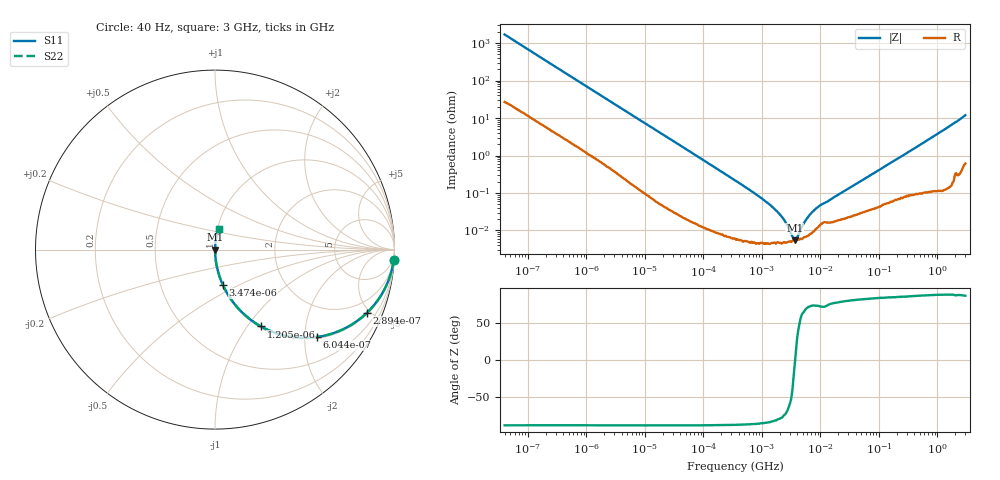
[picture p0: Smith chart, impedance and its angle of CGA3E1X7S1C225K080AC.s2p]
! S-Parameter Data Generated by TDK Corporation
! Copyright(C) 2019 TDK Corporation.
! All Rights Reserved.
! TDK P/N: CGA3E1X7S1C225K080AC (Multilayer Ceramic Chip Capacitor)
! Property: C=2.2uF
! Size(LxWxT): 1.6x0.8x0.8mm
! Model Type: s2p (Touchstone File Format Version 1.0)
! Frequency: DC=Yes Start=4E-05MHz Stop=3000MHz 396points Log-sweep
! Model Generated on July 26, 2019
! Port Assignments:
!  1 ---| |--- 2
! Applicable Conditions:
!  Temperature = 25 degC
!  DC Bias Voltage = 0 V
!  Small Signal Operation
! Terms and conditions regarding TDK Simulation Models
! (1)This simulation model is being provided solely for informational purposes. Please refer to the specifications of the products in terms of detailed characteristics of such products.
! (2)In no event shall TDK Corporation of any of its subsidiaries be liable for any loss or damage arising, directly or indirectly,
!  From any information contained in this simulation model, including, but not limited to loss or damages arising from any inaccuracies, omissions or errors in connection with such information.
! (3)Any and all copyrights on this simulation model are owned by TDK Corporation.
!  Duplication or redistribution of this simulation model without prior written permission from TDK Corporation is prohibited.
! (4)This simulation model is subject to any modification or change without any prior notice.
! (5)Neither TDK Corporation nor any of its subsidiaries shall make any warranty, express or implied,
!  Including but not limited to the correctness, implied warranties of merchantability and fitness for a particular purpose with respect to this simulation models.
! (6)The use of this simulation model shall be deemed to have consented to the terms and conditions hereof.
# Hz S MA R 50
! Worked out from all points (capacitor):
!   395 points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, 40 Hz to 3 GHz, reference 50 ohm
!   read as one part in series: C = 2.34 uF near 41.88 Hz
!   lowest |Z| = 5.48 mohm at 3.622 MHz (marker M1)
!   series resonance near 3.695 MHz, so ESL is about 790 pH
!   S11 on the Smith chart (normalised r, x): 40 Hz: 2, -34; 289.4 Hz: 1.08, -4.77; 604.4 Hz: 1.04, -2.30; 1.205 kHz: 1.02, -1.16; 3.474 kHz: 1.01, -0.41; 3 GHz: 1.01, +0.24
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40  0.9974 -3.4  0.05853 85.7  0.05853 85.7  0.9974 -3.4
138.5867  0.9771 -11.4  0.1972 77.7  0.1972 77.7  0.9771 -11.4
289.415  0.9169 -22.6  0.384 66.5  0.384 66.5  0.9169 -22.6
604.3944  0.7486 -40.6  0.6505 48.5  0.6505 48.5  0.7486 -40.6
834.128  0.6363 -49.5  0.7608 39.5  0.7608 39.5  0.6363 -49.5
1205.403  0.4989 -59.1  0.8584 29.9  0.8584 29.9  0.4989 -59.1
1999.837  0.3311 -69.7  0.9382 19.3  0.9382 19.3  0.3311 -69.7
3474.114  0.2005 -77.6  0.9766 11.6  0.9766 11.6  0.2005 -77.6
7255.102  0.09929 -83.5  0.9937 5.7  0.9937 5.7  0.09929 -83.5
17394.24  0.0423 -86.9  0.9986 2.4  0.9986 2.4  0.0423 -86.9
346410.2  0.002176 -88.3  0.9999 0.1  0.9999 0.1  0.002176 -88.3
1377890  0.0004805 -84.8  1 0.0  1 0.0  0.0004805 -84.8
2286002  0.0002122 -77.2  1 0.0  1 0.0  0.0002122 -77.2
3013016  0.000101 -59.6  0.9999 0.0  0.9999 0.0  0.000101 -59.6
3622024  5.479e-05 -8.9  0.9999 0.0  0.9999 0.0  5.479e-05 -8.9
4559200  0.0001072 55.6  0.9999 -0.0  0.9999 -0.0  0.0001072 55.6
5738865  0.0001982 69.7  0.9999 -0.0  0.9999 -0.0  0.0001982 69.7
7223760  0.0003073 73.6  0.9999 -0.0  0.9999 -0.0  0.0003073 73.6
9969551  0.0004708 72.4  0.9999 -0.0  0.9999 -0.0  0.0004708 72.4
1.506385e8  0.006054 84.5  0.9994 -0.3  0.9994 -0.3  0.006054 84.5
9.940817e8  0.03732 86.2  0.9982 -2.1  0.9982 -2.1  0.03732 86.2
3e9  0.1178 80.3  0.987 -6.8  0.987 -6.8  0.1178 80.3
